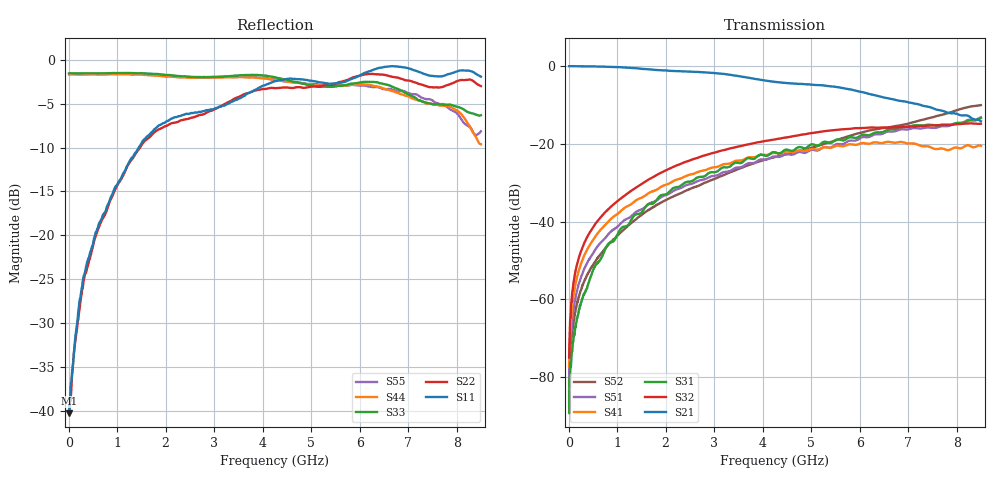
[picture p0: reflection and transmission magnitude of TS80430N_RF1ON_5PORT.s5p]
!Created with skrf (http://scikit-rf.org).
# GHz S RI R 50.0
!freq ReS11 ImS11 ReS12 ImS12 ReS13 ImS13
! ReS14 ImS14 ReS15 ImS15
! ReS21 ImS21 ReS22 ImS22 ReS23 ImS23
! ReS24 ImS24 ReS25 ImS25
! ReS31 ImS31 ReS32 ImS32 ReS33 ImS33
! ReS34 ImS34 ReS35 ImS35
! ReS41 ImS41 ReS42 ImS42 ReS43 ImS43
! ReS44 ImS44 ReS45 ImS45
! ReS51 ImS51 ReS52 ImS52 ReS53 ImS53
! ReS54 ImS54 ReS55 ImS55
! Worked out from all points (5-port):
!   1601 points, 10 MHz to 8.5 GHz, reference 50 ohm
!   strongest paths, dB at 10 MHz, 2.132 GHz, 4.255 GHz, 6.378 GHz, 8.5 GHz:
!     S21: -0.1, -1.3, -4.2, -7.8, -14.2
!     S32: -74.9, -26.1, -18.9, -15.9, -14.9
!     S31: -83.7, -31.6, -22.2, -17.1, -13.4
!     S41: -77.4, -29.8, -22.4, -19.7, -20.6
!     S51: -82.9, -32.3, -23.3, -17.6, -13.2
!     S52: -86.4, -33.7, -23.4, -16.2, -10.1
!   lowest |S11| = -40.3 dB at 15.31 MHz (marker M1), VSWR 1.02, Z = 50.9 - j0.346 ohm
!   |S11| at or under -10 dB: start of sweep to 1.444 GHz
